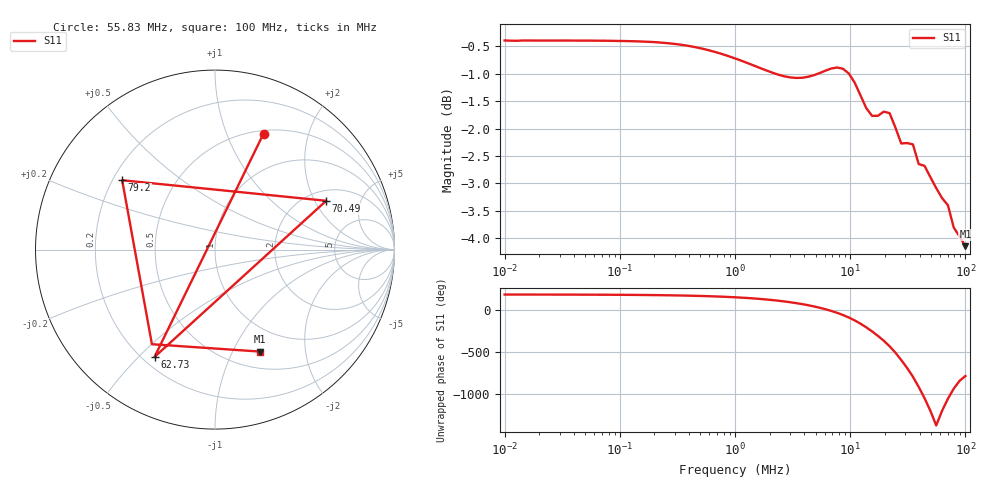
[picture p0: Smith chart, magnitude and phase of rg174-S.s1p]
! ListType=Log
!!RG174 24.9f Short
# MHz S RI R 50
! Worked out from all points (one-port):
!   80 points, 10 kHz to 100 MHz, reference 50 ohm
!   lowest |S11| = -4.1 dB at 100 MHz (marker M1), VSWR 4.28, Z = 34.7 - j64.2 ohm
!   |S11| at or under -10 dB: nowhere
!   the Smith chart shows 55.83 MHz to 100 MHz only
!   S11 on the Smith chart (normalised r, x): 55.83 MHz: 0.53, +1.36; 62.73 MHz: 0.25, -0.56; 70.49 MHz: 2.48, +2.49; 79.2 MHz: 0.24, +0.32; 100 MHz: 0.69, -1.28
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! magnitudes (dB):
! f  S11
! 10 kHz  -0.4
! 32.09 kHz  -0.4
! 103 kHz  -0.4
! 207.2 kHz  -0.4
! 330.4 kHz  -0.5
! 591.8 kHz  -0.6
! 1.06 MHz  -0.7
! 2.397 MHz  -1.0
! 3.401 MHz  -1.1
! 4.294 MHz  -1.1
! 7.693 MHz  -0.9
! 8.644 MHz  -0.9
! 9.713 MHz  -1.0
! 10.91 MHz  -1.2
! 13.78 MHz  -1.6
! 15.48 MHz  -1.8
! 17.4 MHz  -1.8
! 19.55 MHz  -1.7
! 21.97 MHz  -1.7
! 27.74 MHz  -2.3
! 35.02 MHz  -2.3
! 39.35 MHz  -2.6
! 44.21 MHz  -2.7
! 55.83 MHz  -3.1
! 62.73 MHz  -3.3
! 70.49 MHz  -3.4
! 79.2 MHz  -3.8
! 100 MHz  -4.1
